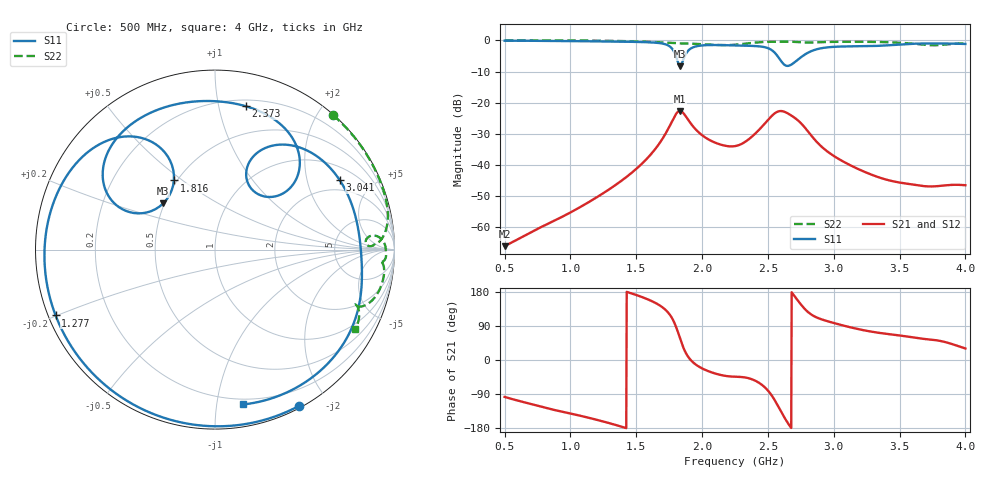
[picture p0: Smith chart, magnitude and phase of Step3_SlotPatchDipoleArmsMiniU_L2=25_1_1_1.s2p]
! TOUCHSTONE file generated by CST MICROWAVE STUDIO
! Date and time: Tue May 19 03:15:05 2020
! Project name: DualBand_DualMode_Antenna_FD_SteppedDesign.cst
! Parameters = {FPL=20; FPW=20; L=50; ST=10; SW=30; W=52; WF=7; ext=10; gap=1; inset=13}
! Header version: 2015
! Port assignment regex: !\s*Touchstone port\s*([0-9]+)\s*=\s*CST MWS port\s*([0-9]+)\s*\(\"(.*)\"\)(\s*mode\s*([0-9]+))?.*
! Touchstone port assignment:
! Touchstone port 1 = CST MWS port 1 ("")
! Touchstone port 2 = CST MWS port 2 ("")
# GHz S MA R 50
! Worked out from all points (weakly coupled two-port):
!   1006 points, 500 MHz to 4 GHz, reference 50 ohm
!   highest |S21| = -22.61 dB at 1.83 GHz (marker M1); lowest = -66.0 dB at 500 MHz (marker M2)
!   lowest |S11| = -8.3 dB at 1.833 GHz (marker M3), VSWR 2.26, Z = 24.6 + j14.9 ohm
!   |S11| at or under -10 dB: nowhere
!   |S22| runs from -1.6 to 0.0 dB; largest |S21 - S12| = 1.1e-05
!   S11 on the Smith chart (normalised r, x): 500 MHz: 0.02, -1.67; 1.277 GHz: 0.02, -0.20; 1.816 GHz: 0.48, +0.46; 2.373 GHz: 0.25, +1.21; 3.041 GHz: 1.51, +3.19; 4 GHz: 0.16, -1.19
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0.5  0.9886 -61.7  0.0005019 -97.4  0.0005019 -97.4  0.9967 48.7
0.787  0.9824 -97.0  0.00104 -124.1  0.001041 -124.1  0.9971 29.4
1.0845  0.9701 -133.7  0.002187 -147.9  0.002188 -147.9  0.9938 18.0
1.277  0.9608 -157.5  0.00387 -164.9  0.003868 -164.9  0.9856 12.5
1.494  0.9462 174.5  0.008482 172.3  0.008482 172.3  0.9636 7.3
1.669  0.9095 147.7  0.02128 146.1  0.02128 146.1  0.9343 4.0
1.7635  0.771 125.3  0.04659 115.2  0.04659 115.2  0.9124 2.6
1.816  0.4481 120.7  0.07168 74.1  0.07168 74.1  0.8986 2.3
1.83  0.3878 134.0  0.07409 59.5  0.07409 59.5  0.8961 2.3
1.8335  0.3866 138.2  0.07406 55.9  0.07406 55.9  0.8956 2.3
1.886  0.6517 153.9  0.05648 13.0  0.05647 13.0  0.8911 2.1
1.935  0.7792 142.8  0.04092 -7.3  0.04092 -7.3  0.8837 1.6
2.25  0.8305 94.7  0.02017 -44.1  0.02017 -44.1  0.8522 4.5
2.3725  0.817 77.8  0.02791 -50.1  0.02791 -50.1  0.9082 4.7
2.5195  0.7189 49.9  0.0586 -89.1  0.0586 -89.1  0.9496 1.0
2.5965  0.4779 39.9  0.07369 -134.0  0.07369 -134.0  0.9524 -0.8
2.705  0.4496 67.3  0.05699 167.1  0.05699 167.1  0.9459 -3.6
2.8345  0.6795 59.2  0.0289 118.9  0.0289 118.9  0.924 -4.1
3.041  0.7954 29.1  0.01244 93.8  0.01243 93.8  0.95 -7.1
3.419  0.8363 -12.0  0.005707 68.3  0.005707 68.3  0.9331 -16.0
3.6605  0.8904 -39.8  0.004672 56.5  0.004672 56.5  0.8602 -21.7
4  0.8768 -79.7  0.00476 30.4  0.004761 30.4  0.8995 -29.6
